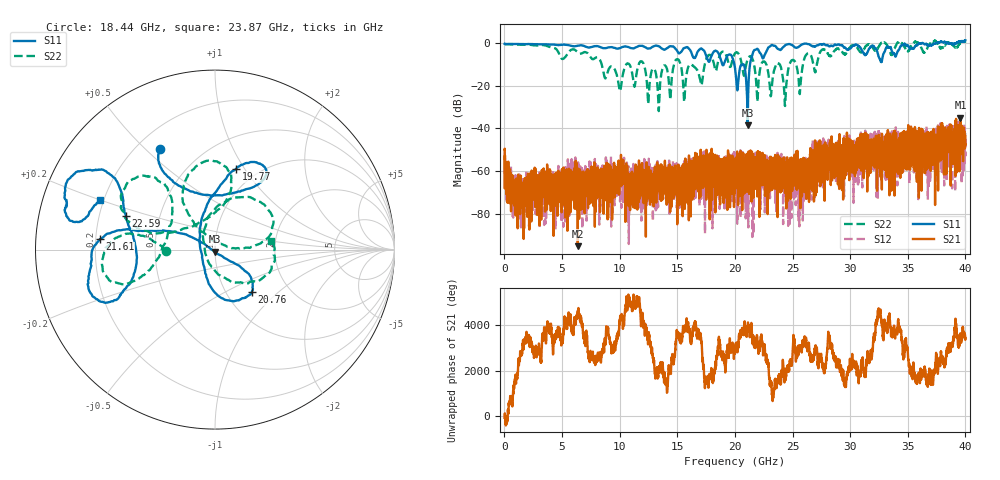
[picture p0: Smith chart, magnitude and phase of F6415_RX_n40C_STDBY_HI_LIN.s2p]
!Keysight Technologies,N5245B,MY52451815,A.15.70.20
!Date: Wednesday, April 17, 2024 15:44:18
!Correction: S33(C  2-Port  )
!S43(C  2-Port  )
!S34(C  2-Port  )
!S44(C  2-Port  )
!S2P File: Measurements: S33, S43, S34, S44:
# Hz S  RI  R 50
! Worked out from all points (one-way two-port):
!   4000 points, 10 MHz to 40 GHz, reference 50 ohm
!   highest |S21| = -34.91 dB at 39.57 GHz (marker M1); lowest = -95.3 dB at 6.36 GHz (marker M2)
!   lowest |S11| = -38.5 dB at 21.1 GHz (marker M3), VSWR 1.02, Z = 49.7 - j1.15 ohm
!   |S11| at or under -10 dB: 18.9 GHz to 19.02 GHz (119.3 MHz wide, 0.629 % of centre); 19.95 GHz to 20.67 GHz (716.2 MHz wide, 3.53 % of centre); 20.75 GHz to 21.31 GHz (561.5 MHz wide, 2.67 % of centre)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
!   |S22| runs from -31.9 to 1.2 dB; largest |S21 - S12| = 0.021
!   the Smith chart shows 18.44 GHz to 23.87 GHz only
!   S11 on the Smith chart (normalised r, x): 18.44 GHz: 0.29, +0.56; 19.77 GHz: 0.80, +0.92; 20.76 GHz: 1.31, -0.69; 21.61 GHz: 0.22, +0.04; 22.59 GHz: 0.32, +0.16; 23.87 GHz: 0.19, +0.20
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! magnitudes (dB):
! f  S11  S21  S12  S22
! 10 MHz  -0.4  -49.9  -51.5  -0.5
! 1.24 GHz  -0.5  -70.2  -64.8  -0.7
! 6.36 GHz  -1.2  -95.3  -60.0  -4.3
! 6.68 GHz  -1.0  -70.8  -57.4  -4.8
! 13.34 GHz  -1.4  -57.7  -69.0  -26.6
! 14.96 GHz  -3.4  -60.8  -77.3  -7.5
! 15.61 GHz  -2.3  -64.1  -59.4  -27.0
! 18.44 GHz  -3.9  -62.6  -57.0  -11.2
! 19.77 GHz  -6.7  -57.4  -74.2  -8.1
! 20.01 GHz  -11.9  -57.5  -55.8  -4.7
! 20.76 GHz  -10.1  -57.4  -65.6  -15.1
! 21.1 GHz  -38.5  -69.8  -80.0  -7.6
! 21.61 GHz  -3.8  -55.4  -64.6  -8.7
! 21.96 GHz  -2.7  -58.6  -55.5  -26.9
! 22.59 GHz  -5.5  -52.5  -79.5  -8.9
! 23.12 GHz  -1.1  -53.4  -58.1  -24.7
! 23.87 GHz  -3.2  -61.5  -59.5  -10.0
! 24.34 GHz  -1.1  -59.8  -66.1  -29.4
! 26.67 GHz  -1.4  -53.7  -53.6  -6.9
! 33.34 GHz  -2.1  -44.2  -41.5  -2.4
! 39.57 GHz  0.8  -34.9  -50.3  0.1
! 40 GHz  1.2  -47.5  -43.8  0.8
